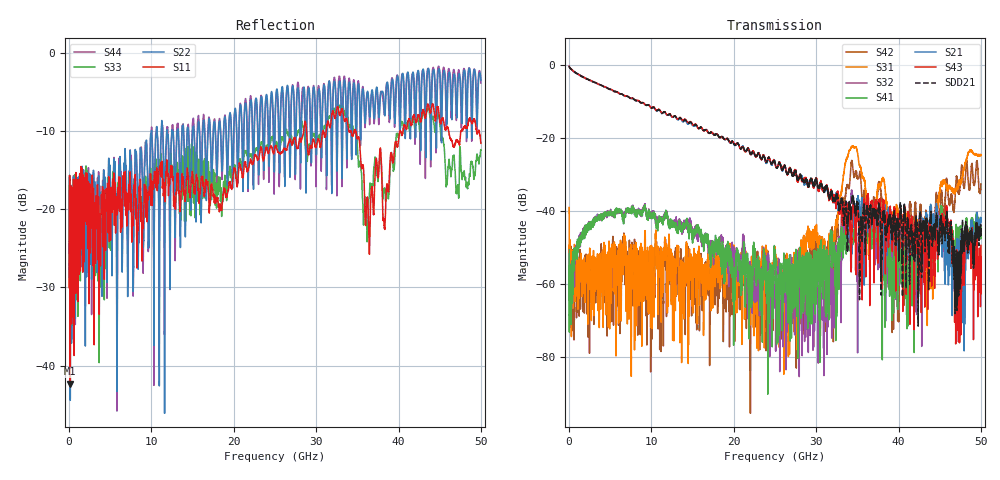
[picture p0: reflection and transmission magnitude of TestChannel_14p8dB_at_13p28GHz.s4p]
# GHz S MA R 50
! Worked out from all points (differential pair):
!   5000 points, 10 MHz to 50 GHz, reference 50 ohm
!   strongest paths, dB at 10 MHz, 12.51 GHz, 25.01 GHz, 37.51 GHz, 50 GHz:
!     S43: -0.3, -14.2, -27.1, -51.9, -49.5
!     S21: -0.3, -14.3, -26.8, -41.5, -43.1
!     S41: -50.6, -42.9, -51.4, -42.9, -47.6
!     S32: -52.4, -43.6, -65.3, -53.4, -45.1
!     S31: -39.1, -51.9, -50.8, -33.4, -24.7
!     S42: -58.2, -57.3, -53.8, -33.6, -32.6
!   taken as a pair (ports 3,1 in; 4,2 out), SDD21 dB: -0.3, -14.2, -26.7, -41.8, -45.2
!   lowest |S11| = -42.3 dB at 150 MHz (marker M1), VSWR 1.02, Z = 49.3 + j0.331 ohm
!   |S11| at or under -10 dB: start of sweep to 28.5 GHz; 28.83 GHz to 30.81 GHz (1.975 GHz wide, 6.62 % of centre); 34.8 GHz to 40.2 GHz (5.4 GHz wide, 14.4 % of centre)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
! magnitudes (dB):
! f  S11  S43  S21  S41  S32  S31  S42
! 10 MHz  -30.0  -0.3  -0.3  -50.6  -52.4  -39.1  -58.2
! 150 MHz  -42.3  -0.8  -0.8  -64.7  -58.7  -60.2  -56.2
! 9.09 GHz  -19.5  -10.5  -10.5  -39.2  -39.3  -57.3  -55.2
! 27.75 GHz  -12.2  -31.7  -31.3  -68.5  -51.3  -66.8  -60.9
! 34.56 GHz  -10.3  -39.6  -43.0  -47.3  -40.3  -22.4  -30.1
! 43.8 GHz  -7.5  -45.1  -40.8  -45.5  -44.2  -56.3  -47.0
! 50 GHz  -11.6  -49.5  -43.1  -47.6  -45.1  -24.7  -32.6
